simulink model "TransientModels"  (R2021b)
settings: Solver=FixedStepAuto  StartTime=0.0  StopTime=10.0  FixedStep=0.0001  RelTol=1e-3
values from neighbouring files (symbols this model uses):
  C_matrix = [Cx_prime*C_sigma/(a*Cx_prime+C_sigma) 0    [ModelComparison.m]
  C_sigma = 3*Fz/sigma_crit    (= 30000)    [ModelComparison.m]    (also in EllipticalContactPatch.m = 33953.0545263; RectangularContactPatch.m = 33953.0545263; CombinedTransientLateralAndCamber.m; NonlinearFullContactPatch.m)
  epsilon = 1*10^(-9)    (= 1e-09)    [ModelComparison.m]    (also in EllipticalContactPatch.m; RectangularContactPatch.m)
  frequency = 0    [ModelComparison.m]
  Fz = 3000    [ModelComparison.m]    (also in EllipticalContactPatch.m; RectangularContactPatch.m; NonlinearFullContactPatch.m)
  initialConditionsF = [Fx0+1*10^(-6); Fy0+1*10^(-6)]    [ModelComparison.m]
  initialConditionsS = [sigma_x0_eq; sigma_y0_eq]    [ModelComparison.m]
  Lambda_inv = [1/lambda_x 0    [ModelComparison.m]
  mu = mu_static    (= 1)    [ModelComparison.m]    (also in CombinedTransientLateralAndCamber.m; NonlinearFullContactPatch.m)
  mu_static = 1    [ModelComparison.m]
  S_prime = [1/Cx_prime 0    [ModelComparison.m]
  sigma = [sigma_x; sigma_y]    [ModelComparison.m]    (also in CombinedTransientLateralAndCamber.m = 0.14; NonlinearFullContactPatch.m = sqrt(sigma_x^2 + sigma_y^2))
libraries: dspmtrx3 x2

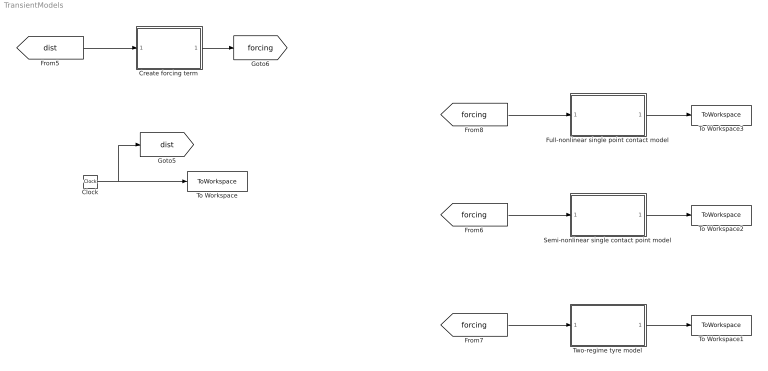
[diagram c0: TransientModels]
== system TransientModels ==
  Clock : Clock
  Create forcing term : Subsystem
  Full-nonlinear single point contact model : Subsystem
  Semi-nonlinear single contact point model : Subsystem
  To Workspace : ToWorkspace  VariableName=distance  SampleTime=-1
  To Workspace1 : ToWorkspace  VariableName=F  SampleTime=-1
  To Workspace2 : ToWorkspace  VariableName=F_single  SampleTime=-1
  To Workspace3 : ToWorkspace  VariableName=F_single_nonlin  SampleTime=-1
  Two-regime tyre model : Subsystem
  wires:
  Clock/1 -> [dist], To Workspace/1
  [dist] -> Create forcing term/1(In1)
  Create forcing term/1(Out1) -> [forcing]
  [forcing] -> Semi-nonlinear single contact point model/1(In1)
  Semi-nonlinear single contact point model/1(Out1) -> To Workspace2/1
  [forcing] -> Two-regime tyre model/1(In1)
  Two-regime tyre model/1(Out1) -> To Workspace1/1
  [forcing] -> Full-nonlinear single point contact model/1(In1)
  Full-nonlinear single point contact model/1(Out1) -> To Workspace3/1

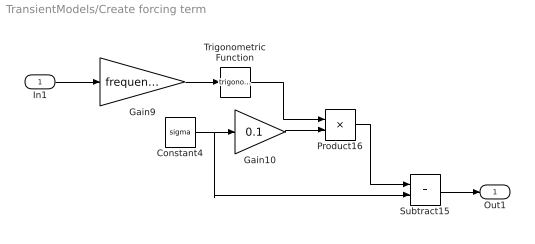
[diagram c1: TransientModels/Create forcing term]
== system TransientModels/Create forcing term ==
  In1 : Inport
  Constant4 : Constant  Value=sigma
  Gain10 : Gain  Gain=0.1
  Gain9 : Gain  Gain=frequency
  Product16 : Product
  Subtract15 : Sum
  Trigonometric Function : Trigonometry
  Out1 : Outport
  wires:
  Subtract15/1 -> Out1/1
  Product16/1 -> Subtract15/1
  Trigonometric Function/1 -> Product16/1
  Gain10/1 -> Product16/2
  In1/1 -> Gain9/1
  Constant4/1 -> Subtract15/2, Gain10/1
  Gain9/1 -> Trigonometric Function/1

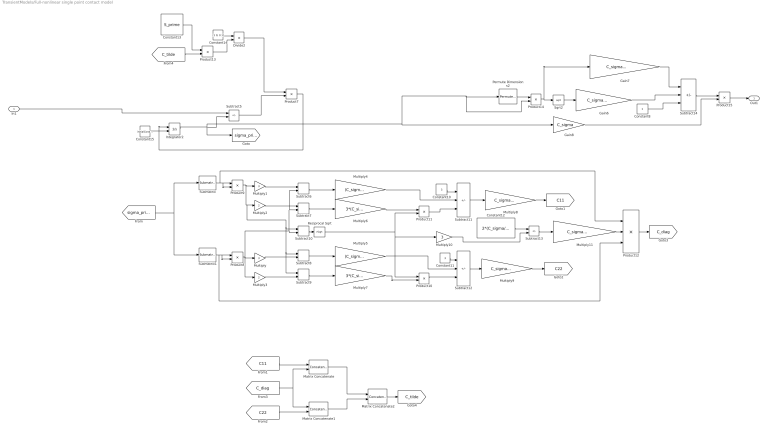
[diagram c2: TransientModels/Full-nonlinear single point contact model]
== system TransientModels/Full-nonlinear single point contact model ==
  In1 : Inport
  Constant10 : Constant  Value=3
  Constant11 : Constant  Value=3
  Constant12 : Constant  Value=2*(C_sigma/(3*mu*Fz))
  Constant13 : Constant  Value=S_prime
  Constant14 : Constant  Value=[1 0; 0 1]
  Constant15 : Constant  Value=initialConditionsS
  Constant8 : Constant
  Divide2 : Product  Inputs=*/  Multiplication=Matrix(*)
  Gain6 : Gain  Gain=C_sigma/(3*mu_static*Fz)
  Gain7 : Gain  Gain=C_sigma^2/(27*(mu_static*Fz)^2)
  Gain8 : Gain  Gain=C_sigma
  Integrator2 : Integrator  InitialConditionSource=external
  Matrix Concatenate : Concatenate  Mode=Multidimensional array  ConcatenateDimension=2
  Matrix Concatenate1 : Concatenate  Mode=Multidimensional array  ConcatenateDimension=2
  Matrix Concatenate2 : Concatenate  Mode=Multidimensional array
  Multiply : Gain  Gain=3
  Multiply1 : Gain  Gain=3
  Multiply10 : Gain  Gain=3
  Multiply11 : Gain  Gain=C_sigma*(C_sigma/(3*mu*Fz))/3
  Multiply2 : Gain  Gain=2
  Multiply3 : Gain  Gain=2
  Multiply4 : Gain  Gain=(C_sigma/(3*mu*Fz))^2
  Multiply5 : Gain  Gain=(C_sigma/(3*mu*Fz))^2
  Multiply6 : Gain  Gain=3*(C_sigma/(3*mu*Fz))
  Multiply7 : Gain  Gain=3*(C_sigma/(3*mu*Fz))
  Multiply8 : Gain  Gain=C_sigma/3
  Multiply9 : Gain  Gain=C_sigma/3
  Permute Dimensions2 : PermuteDimensions
  Product{8..11,15} (5 alike) : Product
  Product12 : Product  Inputs=3
  Product13 : Product  Multiplication=Matrix(*)
  Product14 : Product  Multiplication=Matrix(*)
  Product7 : Product  Multiplication=Matrix(*)
  Reciprocal Sqrt : Sqrt  Operator=rSqrt
  Sqrt2 : Sqrt
  Submatrix : dspmtrx3/Submatrix  RowSpan=One row  RowStartMode=First  RowStartIndex=1  RowEndMode=Last  RowEndIndex=1  ColSpan=Range of columns  ColStartMode=First  ColStartIndex=1  ColEndMode=Last  ColEndIndex=1
  Submatrix1 : dspmtrx3/Submatrix  RowSpan=One row  RowStartMode=Last  RowStartIndex=1  RowEndMode=Last  RowEndIndex=1  ColSpan=Range of columns  ColStartMode=First  ColStartIndex=1  ColEndMode=Last  ColEndIndex=1
  Subtract{6..10} (5 alike) : Sum
  Subtract11 : Sum  Inputs=++-
  Subtract12 : Sum  Inputs=++-
  Subtract13 : Sum  Inputs=+-
  Subtract14 : Sum  Inputs=+-+
  Subtract5 : Sum  Inputs=+-
  Out1 : Outport
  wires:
  Subtract13/1 -> Multiply11/1
  Constant14/1 -> Divide2/1
  Multiply9/1 -> [C22]
  Constant8/1 -> Subtract14/3
  Submatrix/1 -> Product12/1, Product9/2, Product9/1
  Product15/1 -> Out1/1
  Product11/1 -> Subtract11/3
  Product8/1 -> Subtract7/2, Subtract6/2, Subtract10/2, Multiply3/1, Multiply/1
  Subtract10/1 -> Reciprocal Sqrt/1
  Reciprocal Sqrt/1 -> Multiply10/1, Product10/1, Product11/2
  Multiply1/1 -> Subtract6/1
  Product13/1 -> Divide2/2
  Product9/1 -> Subtract8/1, Subtract9/1, Subtract10/1, Multiply2/1, Multiply1/1
  Integrator2/1 -> Product14/2, Permute Dimensions2/1, Gain8/1, [sigma_prime], Subtract5/2
  [C22] -> Matrix Concatenate1/2
  Matrix Concatenate1/1 -> Matrix Concatenate2/2
  Multiply11/1 -> Product12/2
  Constant12/1 -> Subtract13/1
  Multiply6/1 -> Product11/1
  Subtract8/1 -> Multiply5/1
  Subtract5/1 -> Product7/2
  [C_diag] -> Matrix Concatenate1/1, Matrix Concatenate/2
  In1/1 -> Subtract5/1
  Subtract7/1 -> Multiply6/1
  Subtract9/1 -> Multiply7/1
  Multiply7/1 -> Product10/2
  Constant11/1 -> Subtract12/1
  Multiply2/1 -> Subtract7/1
  Gain6/1 -> Subtract14/2
  Constant10/1 -> Subtract11/1
  Product10/1 -> Subtract12/3
  Subtract12/1 -> Multiply9/1
  Product12/1 -> [C_diag]
  Multiply8/1 -> [C11]
  [C_tilde] -> Product13/2
  Multiply10/1 -> Subtract13/2
  Matrix Concatenate2/1 -> [C_tilde]
  Multiply3/1 -> Subtract9/2
  Matrix Concatenate/1 -> Matrix Concatenate2/1
  Constant15/1 -> Integrator2/2
  Permute Dimensions2/1 -> Product14/1
  Subtract14/1 -> Product15/1
  Multiply5/1 -> Subtract12/2
  Submatrix1/1 -> Product12/3, Product8/2, Product8/1
  Product14/1 -> Gain7/1, Sqrt2/1
  Multiply4/1 -> Subtract11/2
  Sqrt2/1 -> Gain6/1
  Constant13/1 -> Product13/1
  Divide2/1 -> Product7/1
  Product7/1 -> Integrator2/1
  Gain8/1 -> Product15/2
  Gain7/1 -> Subtract14/1
  Subtract6/1 -> Multiply4/1
  Subtract11/1 -> Multiply8/1
  Multiply/1 -> Subtract8/2
  [C11] -> Matrix Concatenate/1
  [sigma_prime] -> Submatrix1/1, Submatrix/1

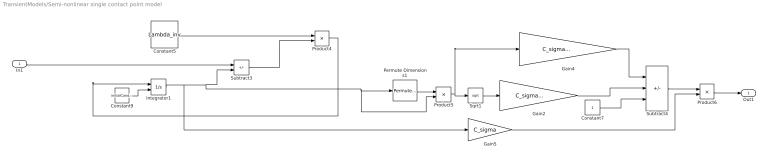
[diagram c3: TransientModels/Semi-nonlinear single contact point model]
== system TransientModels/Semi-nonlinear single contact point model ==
  In1 : Inport
  Constant5 : Constant  Value=Lambda_inv
  Constant7 : Constant
  Constant9 : Constant  Value=initialConditionsS
  Gain2 : Gain  Gain=C_sigma/(3*mu_static*Fz)
  Gain4 : Gain  Gain=C_sigma^2/(27*(mu_static*Fz)^2)
  Gain5 : Gain  Gain=C_sigma
  Integrator1 : Integrator  InitialConditionSource=external
  Permute Dimensions1 : PermuteDimensions
  Product4 : Product  Multiplication=Matrix(*)
  Product5 : Product  Multiplication=Matrix(*)
  Product6 : Product
  Sqrt1 : Sqrt
  Subtract3 : Sum  Inputs=+-
  Subtract4 : Sum  Inputs=+-+
  Out1 : Outport
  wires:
  In1/1 -> Subtract3/1
  Constant9/1 -> Integrator1/2
  Sqrt1/1 -> Gain2/1
  Integrator1/1 -> Gain5/1, Product5/2, Permute Dimensions1/1, Subtract3/2
  Product4/1 -> Integrator1/1
  Subtract3/1 -> Product4/2
  Constant5/1 -> Product4/1
  Product6/1 -> Out1/1
  Subtract4/1 -> Product6/1
  Product5/1 -> Gain4/1, Sqrt1/1
  Gain4/1 -> Subtract4/1
  Gain2/1 -> Subtract4/2
  Constant7/1 -> Subtract4/3
  Gain5/1 -> Product6/2
  Permute Dimensions1/1 -> Product5/1

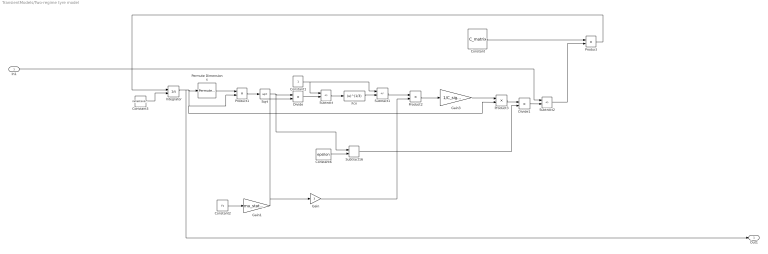
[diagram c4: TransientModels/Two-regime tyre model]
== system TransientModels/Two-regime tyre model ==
  In1 : Inport
  Constant : Constant  Value=C_matrix
  Constant1 : Constant
  Constant2 : Constant  Value=Fz
  Constant3 : Constant  Value=initialConditionsF
  Constant6 : Constant  Value=epsilon
  Divide : Product  Inputs=*/
  Divide1 : Product  Inputs=*/
  Fcn : Fcn  Expr=(u)^(1/3)
  Gain : Gain  Gain=3
  Gain1 : Gain  Gain=mu_static
  Gain3 : Gain  Gain=1/C_sigma
  Integrator : Integrator  InitialConditionSource=external
  Permute Dimensions : PermuteDimensions
  Product : Product  Multiplication=Matrix(*)
  Product1 : Product  Multiplication=Matrix(*)
  Product2 : Product
  Product3 : Product
  Sqrt : Sqrt
  Subtract : Sum  Inputs=+-
  Subtract1 : Sum  Inputs=+-
  Subtract16 : Sum
  Subtract2 : Sum  Inputs=+-
  Out1 : Outport
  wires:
  In1/1 -> Subtract2/1
  Integrator/1 -> Out1/1, Product1/2, Product3/2, Permute Dimensions/1
  Product1/1 -> Sqrt/1
  Gain3/1 -> Product3/1
  Constant/1 -> Product/1
  Permute Dimensions/1 -> Product1/1
  Divide/1 -> Subtract/2
  Subtract/1 -> Fcn/1
  Product/1 -> Integrator/1
  Fcn/1 -> Subtract1/2
  Constant1/1 -> Subtract1/1, Subtract/1
  Constant2/1 -> Gain1/1
  Subtract2/1 -> Product/2
  Divide1/1 -> Subtract2/2
  Subtract16/1 -> Divide1/2
  Product2/1 -> Gain3/1
  Gain1/1 -> Gain/1, Divide/2
  Constant3/1 -> Integrator/2
  Sqrt/1 -> Subtract16/1, Divide/1
  Subtract1/1 -> Product2/1
  Product3/1 -> Divide1/1
  Constant6/1 -> Subtract16/2
  Gain/1 -> Product2/2
